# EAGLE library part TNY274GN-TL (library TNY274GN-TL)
AC/DC Converters 8.5W 85-265 VAC 11W/230 VAC Source: Datasheet
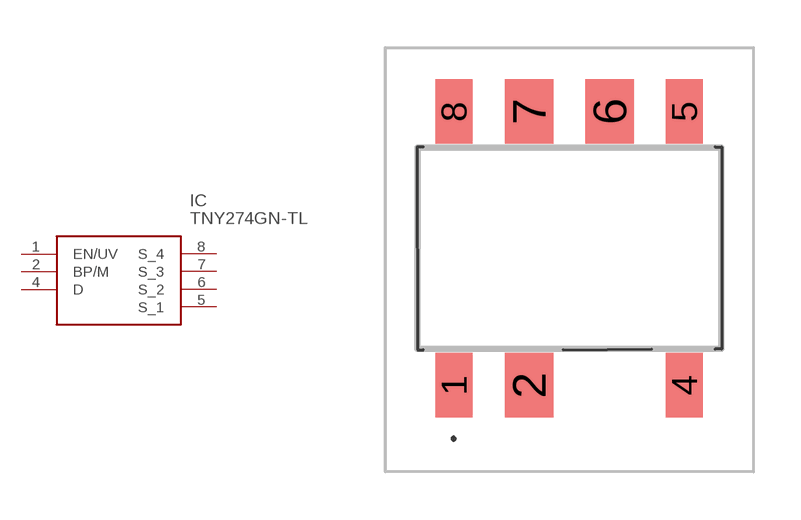
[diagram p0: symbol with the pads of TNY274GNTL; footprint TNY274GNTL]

Designator prefix IC

## TNY274GN-TL (Description: AC/DC Converters 8.5W 85-265 VAC 11W/230 VAC; Height: 3.98mm; Manufacturer_Name: Power Integrations; Manufacturer_Part_Number: TNY274GN-TL; Mouser_Part_Number: 869-TNY274GN-TL; Mouser_Price-Stock: https://www.mouser.co.uk/ProductDetail/Power-Integrations/TNY274GN-TL?qs=%252Bk6%2F5FB6qrlpHJoVM01SMg%3D%3D)  [TNY274GNTL]
1  EN/UV
2  BP/M
4  D
5  S_1
6  S_2
7  S_3
8  S_4

## Footprint TNY274GNTL (pad centres in mm)
TNY274GN-TL-3
smd 1.168 x 2.032: 1 -3.632,-3.452; 4 3.632,-3.452; 5 3.632,5.184; 8 -3.632,5.184
smd 1.524 x 2.032: 2 -1.27,-3.452; 6 1.27,5.184; 7 -1.27,5.184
